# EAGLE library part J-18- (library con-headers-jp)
HEADER JACK PINS
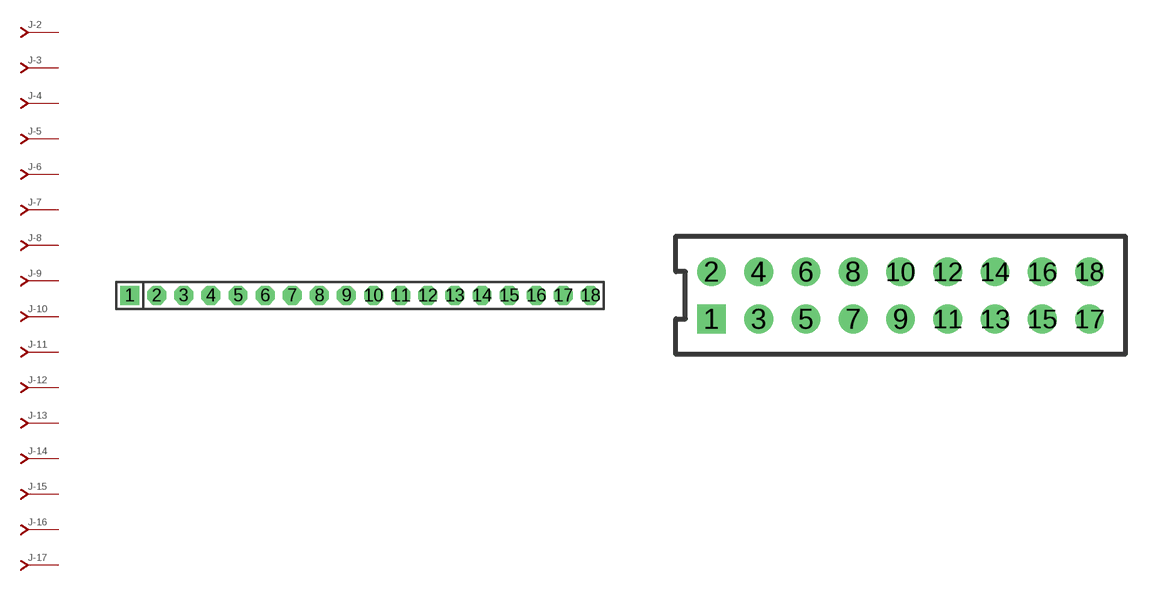
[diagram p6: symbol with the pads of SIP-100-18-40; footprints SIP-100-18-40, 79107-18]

Designator prefix J; gates -2=J-N -3=J-N -4=J-N -5=J-N -6=J-N -7=J-N -8=J-N -9=J-N -10=J-N -11=J-N -12=J-N -13=J-N -14=J-N -15=J-N -16=J-N -17=J-N -18=J-N -1=J-NV

## J-18-SIP-100-40  [SIP-100-18-40]
1  -1:J  pas
2  -2:J  pas
3  -3:J  pas
4  -4:J  pas
5  -5:J  pas
6  -6:J  pas
7  -7:J  pas
8  -8:J  pas
9  -9:J  pas
10  -10:J  pas
11  -11:J  pas
12  -12:J  pas
13  -13:J  pas
14  -14:J  pas
15  -15:J  pas
16  -16:J  pas
17  -17:J  pas
18  -18:J  pas

## J-18-79107  [79107-18]
Pads as for SIP-100-18-40

## J-18-79109  [79109-18]
Pads as for SIP-100-18-40

## J-18-87264  [87264-18]
Pads as for SIP-100-18-40

## J-18-87340  [87340-18]
Pads as for SIP-100-18-40

## J-18-87368  [87368-18]
Pads as for SIP-100-18-40

## J-18-535512  [535512-18]
Pads as for SIP-100-18-40

## J-18-100-2X09  [DIL-100-2X09]
Pads as for SIP-100-18-40

## J-18-100-2X09_M  [DIL-100-2X09_M]
Pads as for SIP-100-18-40

## J-18-2MM-2X09  [DIL-2MM-2X09]
Pads as for SIP-100-18-40

## J-18-2MM-2X09_M  [DIL-2MM-2X09_M]
Pads as for SIP-100-18-40

## J-18-SIP-100-32  [SIP-100-18-32]
Pads as for SIP-100-18-40

## J-18-SIP-100-40Y  [SIP-100-18-40Y]
Pads as for SIP-100-18-40

## J-18-SIP-100-32Y  [SIP-100-18-32Y]
Pads as for SIP-100-18-40

## J-18-71991  [71991-18]
Pads as for SIP-100-18-40

## J-18-KK-4455-B18  [KK-4455-B18]
Pads as for SIP-100-18-40

## J-18-KK-4455-A18  [KK-4455-A18]
Pads as for SIP-100-18-40

## J-18-KK-4455-C18  [KK-4455-C18]
Pads as for SIP-100-18-40

## Footprint SIP-100-18-40 (pad centres in mm)
SIP Header - 0.1", 40 mil drill
drill 1.016 pad 1.778 square: 1 -21.59,0
drill 1.016 pad 1.778 octagon: 2 -19.05,0; 3 -16.51,0; 4 -13.97,0; 5 -11.43,0; 6 -8.89,0; 7 -6.35,0; 8 -3.81,0; 9 -1.27,0; 10 1.27,0; 11 3.81,0; 12 6.35,0; 13 8.89,0; 14 11.43,0; 15 13.97,0; 16 16.51,0; 17 19.05,0; 18 21.59,0

## Footprint 79107-18 (pad centres in mm)
Molex Board-To-Board Receptacal 2.00mm (.079") Pitch Milli-Grid Header, Vertical, Through-Hole Mates with: 87759, 87762, 87758, 87760
drill 0.711 square: 1 -8,-1
drill 0.711: 2 -8,1; 3 -6,-1; 4 -6,1; 5 -4,-1; 6 -4,1; 7 -2,-1; 8 -2,1; 9 0,-1; 10 0,1; 11 2,-1; 12 2,1; 13 4,-1; 14 4,1; 15 6,-1; 16 6,1; 17 8,-1; 18 8,1

## Footprint 79109-18 (pad centres in mm)
Molex Board-to-Board Receptacal 2.00mm (.079") Pitch Milli-Grid Header, Vertical, Top/Bottom Entry Mates with: 87758, 87759, 87760, 87831, 87832, 87833
smd 1.12 x 1.83: 1 -8,-2.65; 2 -8,2.65; 3 -6,-2.65; 4 -6,2.65; 5 -4,-2.65; 6 -4,2.65; 7 -2,-2.65; 8 -2,2.65; 9 0,-2.65; 10 0,2.65; 11 2,-2.65; 12 2,2.65; 13 4,-2.65; 14 4,2.65; 15 6,-2.65; 16 6,2.65; 17 8,-2.65; 18 8,2.65
hole 0.914 at -7,0
hole 0.914 at -8,1
hole 0.914 at -8,-1
hole 0.914 at -6,-1
hole 0.914 at -6,1
hole 0.914 at -4,-1
hole 0.914 at -4,1
hole 0.914 at 7,0
hole 0.914 at -2,1
hole 0.914 at -2,-1
hole 0.914 at 0,1
hole 0.914 at 0,-1
hole 0.914 at 2,1
hole 0.914 at 2,-1
hole 0.914 at 4,1
hole 0.914 at 4,-1
hole 0.914 at 6,-1
hole 0.914 at 6,1
hole 0.914 at 8,1
hole 0.914 at 8,-1

## Footprint 87264-18 (pad centres in mm)
Molex Board-To-Board Receptacal 2.00mm (.079") Pitch Milli-Grid Header, Side Entry Mates with 2mm(.079") Mill-Grid Header
drill 0.914 square: 1 -8,-2.25
drill 0.914: 2 -8,2.25; 3 -6,-2.25; 4 -6,2.25; 5 -4,-2.25; 6 -4,2.25; 7 -2,-2.25; 8 -2,2.25; 9 0,-2.25; 10 0,2.25; 11 2,-2.25; 12 2,2.25; 13 4,-2.25; 14 4,2.25; 15 6,-2.25; 16 6,2.25; 17 8,-2.25; 18 8,2.25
